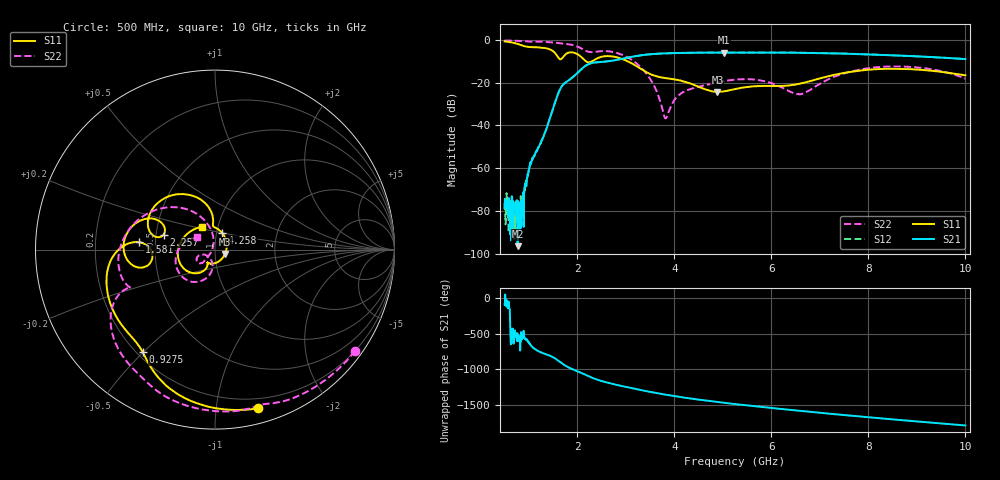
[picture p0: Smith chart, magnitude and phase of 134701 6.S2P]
!  2-Port S-parameters saved by WinCal
! VAR MeasName=S-Parameters (CALIBRATED_DATA) read from VNA (N5242A)
! VAR MeasDate=2013-7-3 16:22:04
! VAR NAME=134701 6
! VAR FILENAME=134701 6.S2P
! VAR DATE=2013-7-3 16:22:04
! VAR PHYS_PORTS=1,2
# Hz S MA R 50
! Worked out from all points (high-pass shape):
!   1601 points, 500 MHz to 10 GHz, reference 50 ohm
!   highest |S21| = -5.99 dB at 5.03 GHz (marker M1); lowest = -96.4 dB at 767.2 MHz (marker M2)
!   |S21| within 3 dB of the highest: 2.897 GHz to 9.983 GHz (7.087 GHz wide, 110 % of centre)
!   lowest |S11| = -24.3 dB at 4.888 GHz (marker M3), VSWR 1.13, Z = 55.8 - j2.7 ohm
!   |S11| at or under -10 dB: 2.174 GHz to 2.309 GHz (134.9 MHz wide, 6.02 % of centre); 3.034 GHz to end of sweep
!   |S22| runs from -36.7 to -0.3 dB; largest |S21 - S12| = 0.0022
!   S11 on the Smith chart (normalised r, x): 500 MHz: 0.12, -1.30; 927.5 MHz: 0.22, -0.50; 1.581 GHz: 0.40, +0.04; 2.257 GHz: 0.55, +0.10; 4.258 GHz: 1.06, +0.20; 10 GHz: 0.83, +0.22
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5e8  0.9171 -74.8  0.0001163 -90.2  0.0001543 -95.0  0.9631 -35.9
7.671875e8  0.8001 -110.5  1.519e-05 -136.3  7.169e-05 149.7  0.9455 -54.9
8.503125e8  0.7421 -119.2  0.0001225 164.4  9.689e-05 -169.7  0.9372 -60.9
9.275e8  0.6993 -125.2  0.0003668 148.6  0.0003941 139.9  0.9248 -66.4
1.034375e9  0.6743 -132.5  0.001223 60.2  0.001265 63.2  0.9027 -73.0
1.372812e9  0.6277 -164.3  0.009029 -72.4  0.009037 -73.1  0.8895 -97.2
1.580625e9  0.4243 174.4  0.04708 -142.5  0.04701 -142.7  0.8464 -113.3
2.085312e9  0.3913 153.7  0.2079 31.0  0.207 30.9  0.6259 -153.0
2.2575e9  0.2984 163.7  0.2779 -21.6  0.2769 -21.7  0.5174 -155.7
2.61375e9  0.4154 148.4  0.3125 -102.8  0.3116 -102.8  0.5419 -173.8
3.106562e9  0.2876 105.6  0.3971 -178.9  0.3967 -178.7  0.3481 137.3
3.670625e9  0.1361 94.7  0.4739 105.3  0.4729 105.3  0.0493 99.2
3.825e9  0.1268 93.2  0.4817 87.1  0.4818 87.2  0.01481 166.5
4.258438e9  0.1013 66.6  0.495 41.7  0.4944 41.8  0.06608 -134.9
4.887812e9  0.06067 -23.4  0.5007 -14.6  0.501 -14.6  0.101 -133.7
5.030312e9  0.06287 -47.4  0.502 -26.3  0.5016 -26.2  0.1085 -135.5
5.25e9  0.07051 -76.3  0.5009 -43.6  0.5014 -43.6  0.1173 -140.1
5.998125e9  0.08345 -119.3  0.5005 -97.9  0.5002 -97.9  0.09718 -159.8
6.538438e9  0.09175 -116.6  0.4984 -134.9  0.4982 -134.9  0.0539 -135.1
6.835312e9  0.1109 -115.1  0.4941 -154.6  0.4942 -154.5  0.07155 -103.0
8.420625e9  0.2103 -161.3  0.4372 107.6  0.4358 107.5  0.2376 -141.2
1e10  0.1479 120.5  0.3547 17.9  0.354 18.0  0.1233 145.2
